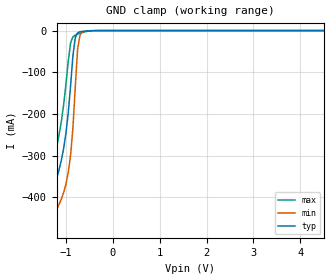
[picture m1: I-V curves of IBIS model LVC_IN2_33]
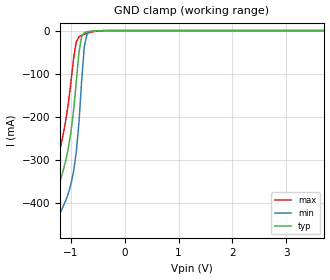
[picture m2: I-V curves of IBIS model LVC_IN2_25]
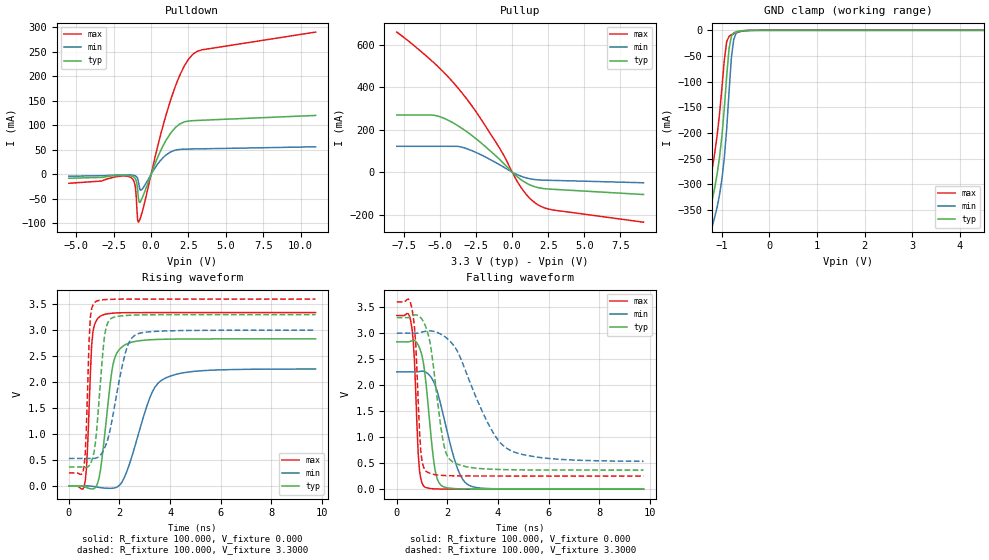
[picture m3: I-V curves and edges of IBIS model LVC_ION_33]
| NXP Semiconductors
| Logic Products Group
| IBIS model of 74LVC245A
|  OCTAL BUS TRANSCEIVER WITH DIRECTION PIN; 3-STATE; 5V TOLERANT
|[Packages]:
|[Package1]: SO 20-pin (D) Package ;
|[Package2]: SSOP 20-Pin Packages ;
|[Package3]: TSSOP 20-pin (PW) Package ;
|[Package4]: DHVQFN 20-pin (BQ) Package ;
[IBIS Ver]   3.2
[File Name]   lvc245a.ibs
[File Rev]   1.4
[Date]   06-Apr-2012
[Source]   File created from simulations by LPG
   NXP Semiconductors Nijmegen
[Notes]   V1.4   Ibis model.
| Remark:
| The Power Clamp curves have been omitted since there is no power clamp diode.
| Revision History
| Version Date   Author/ Description
|   Editor
| 1.0   1999   Initial Version
| 1.1   November 2001 RM   Revised for Ibis 3.2:
|   Added Model Spec and Model Selector
| 1.2   April   2002 RM   Corrected Model mapping in package models
| 1.3   November 2002 RM   Revised: Power Clamp curves omitted, constant
|   end points for Ground Clamp and V/t curves.
| 1.4   April   2012 RV   Updates pcakge models.
|   Added DHVQFN (BQ) package model
[Disclaimer]
   NXP Semiconductors warrants and represents that the IBIS model
   identified herein is owned by NXP Semiconductors (NXP). The
   model provided is not warranted as fully representing all of the
   operating characteristics and specifications of the semiconductor
   products to which the model relates.  Moreover, unless there is a
   signed, written agreement to the contrary, this IBIS model is
   furnished on an "as is" basis without support or warranty of any
   kind, either expressed or implied, regarding the use thereof, and
   NXP specifically disclaims all implied warranties of
   merchantability and fitness of the model for any purpose.
   NXP does not assume any liability arising out of the application
   or use of this IBIS model including infringement of patents and
   copyrights, nor does NXP convey any license under its patents and
   copyrights or the rights of others.
   NXP provides IBIS models as a service to our customers. You and
   your company shall not distribute, convey, sell, or give these models
   to anyone else without receiving prior written permission from
   NXP.
   NXP reserves the right to make changes without notice to these
   IBIS models to improve reliability, function, or design.
   Please be aware that your receipt and subsequent use of the IBIS
   information provided shall serve as acceptance of the terms and
   conditions of this agreement.  If you do not accept these terms,
   you should return or destroy the IBIS models and any other
   accompanying information immediately.
[Copyright]
   (C) Copyright 2012 NXP Semiconductors
   All rights reserved
|   Info for  SO 20-pin (D) Package
[Component]   74LVC245A_D
[Manufacturer]   NXP Semiconductors
[Package]
|   typ   min   max
R_pkg   1.303E-01   1.269E-01   1.360E-01
L_pkg   4.335E-09   3.559E-09   5.739E-09
C_pkg   8.078E-13   6.647E-13   1.016E-12
[Pin] signal_name   model_name   R_pin   L_pin   C_pin
   1   DIR   lvc_in2 1.359E-01   5.726E-09   1.016E-12
   2   A0   lvc_ion 1.318E-01   4.676E-09   8.893E-13
   3   A1   lvc_ion 1.290E-01   3.989E-09   7.599E-13
   4   A2   lvc_ion 1.277E-01   3.713E-09   7.096E-13
   5   A3   lvc_ion 1.269E-01   3.565E-09   6.651E-13
   6   A4   lvc_ion 1.269E-01   3.566E-09   6.652E-13
   7   A5   lvc_ion 1.278E-01   3.720E-09   7.096E-13
   8   A6   lvc_ion 1.291E-01   4.009E-09   7.592E-13
   9   A7   lvc_ion 1.319E-01   4.689E-09   8.893E-13
   10   GND   GND 1.359E-01   5.726E-09   1.016E-12
   11   B7   lvc_ion 1.360E-01   5.739E-09   1.015E-12
   12   B6   lvc_ion 1.319E-01   4.687E-09   8.894E-13
   13   B5   lvc_ion 1.289E-01   3.979E-09   7.598E-13
   14   B4   lvc_ion 1.277E-01   3.706E-09   7.097E-13
   15   B3   lvc_ion 1.269E-01   3.560E-09   6.648E-13
   16   B2   lvc_ion 1.269E-01   3.559E-09   6.647E-13
   17   B1   lvc_ion 1.277E-01   3.707E-09   7.096E-13
   18   B0   lvc_ion 1.290E-01   3.990E-09   7.589E-13
   19   OE#   lvc_in2 1.318E-01   4.674E-09   8.891E-13
   20   VCC   POWER 1.359E-01   5.719E-09   1.016E-12
|   Info for SSOP (DB) 20-Pin Packages
[Component]   74LVC245A_DB
[Manufacturer]   NXP Semiconductors
[Package]
|   typ   min   max
R_pkg   1.170E-01   9.466E-02   1.330E-01
L_pkg   2.881E-09   2.301E-09   3.694E-09
C_pkg   5.134E-13   4.076E-13   6.074E-13
[Pin] signal_name   model_name   R_pin   L_pin   C_pin
   1   DIR   lvc_in2 1.319E-01   3.694E-09   5.788E-13
   2   A0   lvc_ion 1.294E-01   3.215E-09   6.058E-13
   3   A1   lvc_ion 1.259E-01   2.779E-09   5.353E-13
   4   A2   lvc_ion 1.028E-01   2.436E-09   4.753E-13
   5   A3   lvc_ion 9.475E-02   2.308E-09   4.565E-13
   6   A4   lvc_ion 9.474E-02   2.307E-09   4.568E-13
   7   A5   lvc_ion 1.028E-01   2.433E-09   4.753E-13
   8   A6   lvc_ion 1.259E-01   2.774E-09   5.356E-13
   9   A7   lvc_ion 1.295E-01   3.206E-09   6.070E-13
   10   GND   GND 1.330E-01   3.679E-09   4.076E-13
   11   B7   lvc_ion 1.317E-01   3.678E-09   5.790E-13
   12   B6   lvc_ion 1.293E-01   3.209E-09   6.060E-13
   13   B5   lvc_ion 1.258E-01   2.758E-09   5.351E-13
   14   B4   lvc_ion 1.028E-01   2.427E-09   4.749E-13
   15   B3   lvc_ion 9.466E-02   2.301E-09   4.565E-13
   16   B2   lvc_ion 9.472E-02   2.307E-09   4.566E-13
   17   B1   lvc_ion 1.028E-01   2.434E-09   4.750E-13
   18   B0   lvc_ion 1.259E-01   2.769E-09   5.354E-13
   19   OE#   lvc_in2 1.296E-01   3.220E-09   6.074E-13
   20   VCC   POWER 1.329E-01   3.680E-09   4.076E-13
|   Info for  TSSOP 20-pin (PW) Package
[Component]   74LVC245A_PW
[Manufacturer]   NXP Semiconductors
[Package]
|   typ   min   max
R_pkg   8.765E-02   8.574E-02   9.134E-02
L_pkg   2.180E-09   1.913E-09   2.812E-09
C_pkg   3.300E-13   2.758E-13   4.019E-13
[Pin] signal_name   model_name   R_pin   L_pin   C_pin
   1   DIR   lvc_in2 9.132E-02   2.811E-09   4.003E-13
   2   A0   lvc_ion 8.924E-02   2.335E-09   3.938E-13
   3   A1   lvc_ion 8.600E-02   1.921E-09   2.996E-13
   4   A2   lvc_ion 8.597E-02   1.922E-09   2.800E-13
   5   A3   lvc_ion 8.576E-02   1.914E-09   2.764E-13
   6   A4   lvc_ion 8.574E-02   1.913E-09   2.767E-13
   7   A5   lvc_ion 8.595E-02   1.921E-09   2.803E-13
   8   A6   lvc_ion 8.594E-02   1.921E-09   2.995E-13
   9   A7   lvc_ion 8.925E-02   2.334E-09   3.943E-13
   10   GND   GND 9.130E-02   2.809E-09   4.019E-13
   11   B7   lvc_ion 9.134E-02   2.812E-09   4.002E-13
   12   B6   lvc_ion 8.925E-02   2.332E-09   3.937E-13
   13   B5   lvc_ion 8.600E-02   1.920E-09   2.993E-13
   14   B4   lvc_ion 8.597E-02   1.921E-09   2.794E-13
   15   B3   lvc_ion 8.576E-02   1.914E-09   2.758E-13
   16   B2   lvc_ion 8.574E-02   1.913E-09   2.762E-13
   17   B1   lvc_ion 8.596E-02   1.921E-09   2.798E-13
   18   B0   lvc_ion 8.595E-02   1.921E-09   2.993E-13
   19   OE#   lvc_in2 8.925E-02   2.331E-09   3.936E-13
   20   VCC   POWER 9.134E-02   2.812E-09   4.003E-13
|   Info for  DHVQFN 20-pin (BQ) Package
[Component]   74LVC245A_BQ
[Manufacturer]   NXP Semiconductors
[Package]
|   typ   min   max
R_pkg   9.848E-02   7.975E-02   1.188E-01
L_pkg   1.518E-09   1.230E-09   1.831E-09
C_pkg   2.028E-13   1.724E-13   2.307E-13
[Pin] signal_name   model_name   R_pin   L_pin   C_pin
   1   DIR   lvc_in2 1.187E-01   1.831E-09   2.169E-13
   2   A0   lvc_ion 1.188E-01   1.831E-09   2.166E-13
   3   A1   lvc_ion 9.536E-02   1.470E-09   2.030E-13
   4   A2   lvc_ion 7.977E-02   1.230E-09   1.851E-13
   5   A3   lvc_ion 7.977E-02   1.230E-09   1.851E-13
   6   A4   lvc_ion 7.977E-02   1.230E-09   1.849E-13
   7   A5   lvc_ion 7.977E-02   1.230E-09   1.851E-13
   8   A6   lvc_ion 9.536E-02   1.470E-09   2.028E-13
   9   A7   lvc_ion 1.188E-01   1.830E-09   2.300E-13
   10   GND   GND 1.188E-01   1.830E-09   2.307E-13
   11   B7   lvc_ion 1.188E-01   1.831E-09   2.173E-13
   12   B6   lvc_ion 1.187E-01   1.831E-09   2.168E-13
   13   B5   lvc_ion 9.534E-02   1.471E-09   1.902E-13
   14   B4   lvc_ion 7.975E-02   1.231E-09   1.724E-13
   15   B3   lvc_ion 7.977E-02   1.230E-09   1.857E-13
   16   B2   lvc_ion 7.977E-02   1.230E-09   1.850E-13
   17   B1   lvc_ion 7.975E-02   1.230E-09   1.849E-13
   18   B0   lvc_ion 9.535E-02   1.470E-09   2.029E-13
   19   OE#   lvc_in2 1.188E-01   1.830E-09   2.301E-13
   20   VCC   POWER 1.188E-01   1.830E-09   2.299E-13
[Model Selector]   lvc_in2
LVC_IN2_33   3.3V-Vcc input model
LVC_IN2_25   2.5V-Vcc input model
[Model Selector]   lvc_ion
LVC_ION_33   3.3V-Vcc I/O model, non-inverting
LVC_ION_25   2.5V-Vcc I/O model, non-inverting
| Models and submodels in the file (4): LVC_IN2_33 (Input), LVC_IN2_25 (Input), LVC_ION_33 (I/O), LVC_ION_25 (I/O)
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| Remark: If your software does not support the Model Selector
|   Please comment out the lines of the Model Selector, which
|   contain the name of the Model, except the one you want to use.
|   Model LVC_IN2_33
[Model]   LVC_IN2_33
Model_type   Input
Vinl =   0.8000V
Vinh =   2.0000V
C_comp   2.78pF   1.99pF   3.72pF
[Model Spec]
| Note: The input and output voltage ratings may be exceeded if the input and
|   output current ratings are observed (please refer to the data sheet)
|   Subparameter   typ   min   max
| Thresholds
Vinh   2.0   NA   NA
Vinl   0.8   NA   NA
| Overshoot
S_overshoot_high   6.5   6.5   6.5   | Static overshoot
S_overshoot_low   -0.5   -0.5   -0.5
D_overshoot_high   7.2   7.2   7.2   | Dynamic overshoot
D_overshoot_low   -0.95   -0.9   -1.0
D_overshoot_time   3n   3n   3n
|Ambient temperature:   25.0000   85.0000   -40.0000
[Temperature Range]   40.0000   100.0000   -25.0000
[Voltage Range]   3.3000V   3.0000V   3.6000V
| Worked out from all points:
|   GND clamp passes 1 mA (typ) near -0.57 V on its own axis
|Process Range   nominal   slow   fast
[GND_clamp]
| voltage   I(typ)   I(min)   I(max)
-5.5V     -4.567A    -4.624A    -4.51A
-1.45V    -555.2mA   -621.5mA   -488.4mA
-1.35V    -461.8mA   -528.7mA   -394.3mA
-1.3V     -417.5mA   -485mA     -349.4mA
-1.1V     -312.4mA   -404.8mA   -219.8mA
-950mV    -197.3mA   -340.4mA   -73.13mA
-900mV    -132mA     -298.5mA   -29.44mA
-850mV    -59.79mA   -233mA     -14.94mA
-800mV    -16.87mA   -135mA     -10.93mA
-750mV    -5.479mA   -44.49mA   -8.487mA
-700mV    -2.88mA    -11.01mA   -6.407mA
5.5V      1.567nA    9.324nA    202.5pA
|   Model LVC_IN2_25
[Model]   LVC_IN2_25
Model_type   Input
Vinl =   0.7000V
Vinh =   1.7000V
C_comp   2.84pF   2.10pF   3.71pF
[Model Spec]
| Note: The input and output voltage ratings may be exceeded if the input and
|   output current ratings are observed (please refer to the data sheet)
|   Subparameter   typ   min   max
| Thresholds
Vinh   1.7   NA   NA
Vinl   0.7   NA   NA
| Overshoot
S_overshoot_high   6.5   6.5   6.5   | Static overshoot
S_overshoot_low   -0.5   -0.5   -0.5
D_overshoot_high   7.2   7.2   7.2   | Dynamic overshoot
D_overshoot_low   -0.95   -0.9   -1.0
D_overshoot_time   3n   3n   3n
|Ambient temperature:   25.0000   85.0000   -40.0000
[Temperature Range]   35.0000   95.0000   -30.0000
[Voltage Range]   2.5000V   2.3000V   2.7000V
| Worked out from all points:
|   GND clamp passes 1 mA (typ) near -0.57 V on its own axis
|Process Range   nominal   slow   fast
[GND_clamp]
| voltage   I(typ)   I(min)   I(max)
-5.5V     -4.558A    -4.615A    -4.502A
-1.45V    -549mA     -615mA     -482.5mA
-1.35V    -455.6mA   -522.2mA   -388.4mA
-1.3V     -411.3mA   -478.6mA   -343.5mA
-1.1V     -304mA     -396mA     -212mA
-950mV    -185.1mA   -326.6mA   -65.02mA
-900mV    -119.1mA   -281.8mA   -26.08mA
-850mV    -50.24mA   -213.2mA   -14.46mA
-800mV    -13.81mA   -116mA     -10.88mA
-750mV    -4.865mA   -35.92mA   -8.446mA
-700mV    -2.732mA   -8.828mA   -6.333mA
5.5V      922.9pA    6.4nA      86.94pA
|   Model LVC_ION_33
[Model]   LVC_ION_33
Model_type   I/O
Polarity   Non-Inverting
Enable   Active-Low
Vinl  =  0.8000V
Vinh  =  2.0000V
Vmeas =  1.5000V
Cref  = 50.0000pF
Rref  =  0.5000k
Vref  =  0.000V
C_comp   3.67pF   3.24pF   4.23pF
[Model Spec]
| Note: The input and output voltage ratings may be exceeded if the input and
|   output current ratings are observed (please refer to the data sheet)
|   Subparameter   typ   min   max
| Overshoot
S_overshoot_high   6.5   6.5   6.5   | Static overshoot
S_overshoot_low   -0.5   -0.5   -0.5
D_overshoot_high   7.2   7.2   7.2   | Dynamic overshoot
D_overshoot_low   -0.95   -0.9   -1.0
D_overshoot_time   3n   3n   3n
| Timing Thresholds
Vmeas   1.5   1.5   1.5
|Ambient temperature:   25.0000   85.0000   -40.0000
[Temperature Range]   40.0000   100.0000   -25.0000
[Voltage Range]   3.3000V   3.0000V   3.6000V
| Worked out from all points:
|   slope of the pulldown table from 0 to 0.495 V, typ, clamps not added: 12.8 ohm
|   slope of the pullup table from 0 to 0.495 V, typ, clamps not added: 16.7 ohm
|   GND clamp passes 1 mA (typ) near -0.57 V on its own axis
|   rising waveform, R_fixture 100.000, V_fixture 0.000: 20-80 % time 400ps typ, 877ps min, 167ps max; typ from 0 V to 2.83 V
|   rising waveform, R_fixture 100.000, V_fixture 3.3000: 20-80 % time 297ps typ, 599ps min, 140ps max; typ from 0.367 V to 3.3 V
|   falling waveform, R_fixture 100.000, V_fixture 0.000: 20-80 % time 354ps typ, 719ps min, 176ps max; typ from 2.83 V to 0 V
|   falling waveform, R_fixture 100.000, V_fixture 3.3000: 20-80 % time 471ps typ, 1.35ns min, 197ps max; typ from 3.3 V to 0.367 V
|Process Range   nominal   slow   fast
[Pulldown]
| voltage   I(typ)   I(min)   I(max)
-5.5V     -7.981mA   -3.814mA   -18.26mA
-1.35V    -3.285mA   -1.337mA   -6.644mA
-1.05V    -9.131mA   -3.158mA   -26.89mA
-900mV    -31.33mA   -8.405mA   -93.71mA
-850mV    -48.34mA   -14.32mA   -97.69mA
-800mV    -56.89mA   -23.68mA   -95.44mA
-650mV    -51.7mA    -31.9mA    -82.65mA
500mV     38.92mA    23.46mA    64.5mA
1.3V      83.8mA     45.64mA    151.3mA
2.2V      106.9mA    51.35mA    220.1mA
2.8V      109.6mA    51.79mA    245.4mA
11V       120.3mA    56.22mA    290.4mA
[Pullup]
| voltage   I(typ)   I(min)   I(max)
-8V       269.1mA    121.8mA    660.4mA
-5.4V     268mA      121.8mA    514mA
-4.4V     243.3mA    121.8mA    446.3mA
-3.6V     211.5mA    119.5mA    383.9mA
-2.4V     151.5mA    89.4mA     274mA
-800mV    55.11mA    31.81mA    104.4mA
600mV     -35.22mA   -19.02mA   -71.23mA
1V        -52.59mA   -27.82mA   -107.4mA
1.6V      -69.81mA   -35.37mA   -146mA
2.2V      -77.8mA    -37.89mA   -167.8mA
2.8V      -81.05mA   -39.02mA   -178.1mA
9.1V      -105.6mA   -50.26mA   -236.2mA
[GND_clamp]
| voltage   I(typ)   I(min)   I(max)
-5.5V     -4.552A    -4.581A    -4.529A
-1.35V    -436.9mA   -483.2mA   -382.8mA
-1.3V     -392.7mA   -439.6mA   -337.9mA
-1.2V     -328.9mA   -381mA     -268.2mA
-1.05V    -247.4mA   -320.5mA   -163.3mA
-950mV    -153.3mA   -249mA     -58.72mA
-900mV    -90.37mA   -192.9mA   -22.55mA
-850mV    -36.04mA   -120.8mA   -11.79mA
-800mV    -11.48mA   -52.5mA    -8.579mA
-750mV    -4.615mA   -17.21mA   -6.53mA
-700mV    -2.665mA   -5.464mA   -4.804mA
5.5V      991.5pA    8.054nA    37.33pA
[Ramp]
| variable   typ   min   max
dV/dt_r   1.700V/400.499ps   1.352V/877.029ps   2.004V/166.817ps
dV/dt_f   1.760V/471.272ps   1.479V/1.352ns   2.008V/196.882ps
R_load = 100.000
[Rising Waveform]
R_fixture   = 100.000
V_fixture   = 0.000
V_fixture_min = 0.000
V_fixture_max = 0.000
| time   V(typ)   V(min)   V(max)
0s        66.72pV    2.831nV    5.104pV
650ps     -20.04mV   787uV      106.7mV
750ps     -38.64mV   1.118mV    865.9mV
900ps     -55.77mV   -3.748mV   2.705V
1.25ns    312.5mV    -31.4mV    3.272V
1.75ns    2.35V      -42.26mV   3.329V
2.2ns     2.713V     172.1mV    3.337V
3.2ns     2.816V     1.7V       3.34V
3.7ns     2.825V     2.047V     3.34V
9.75ns    2.833V     2.253V     3.34V
[Rising Waveform]
R_fixture   = 100.000
V_fixture   = 3.3000
V_fixture_min = 3.0000
V_fixture_max = 3.6000
| time   V(typ)   V(min)   V(max)
0s        366.8mV    531.4mV    252.7mV
600ps     358.5mV    532mV      365.8mV
650ps     356.5mV    532.2mV    639.8mV
850ps     427.8mV    529.9mV    3.253V
1.05ns    835.2mV    534.7mV    3.548V
1.4ns     2.845V     722.3mV    3.588V
1.7ns     3.235V     1.252V     3.596V
2.25ns    3.284V     2.593V     3.599V
2.7ns     3.293V     2.925V     3.6V
9.75ns    3.3V       3V         3.6V
[Falling Waveform]
R_fixture   = 100.000
V_fixture   = 0.000
V_fixture_min = 0.000
V_fixture_max = 0.000
| time   V(typ)   V(min)   V(max)
0s        2.833V     2.255V     3.34V
550ps     2.845V     2.255V     3.241V
700ps     2.855V     2.254V     2.457V
900ps     2.715V     2.264V     349.4mV
1.1ns     2.269V     2.259V     43.59mV
1.5ns     408.7mV    2.02V      5.848mV
1.8ns     57.88mV    1.501V     2.421mV
2.4ns     8.231mV    399.2mV    587.4uV
2.95ns    3.443mV    54.81mV    163.2uV
9.75ns    -682.6nV   100.1uV    3.08pV
[Falling Waveform]
R_fixture   = 100.000
V_fixture   = 3.3000
V_fixture_min = 3.0000
V_fixture_max = 3.6000
| time   V(typ)   V(min)   V(max)
0s        3.3V       3V         3.6V
600ps     3.326V     2.999V     3.473V
750ps     3.353V     2.998V     2.782V
950ps     3.295V     3.014V     728.3mV
1.15ns    3.116V     3.038V     345.8mV
1.35ns    2.716V     3.043V     298.4mV
1.85ns    878.2mV    2.95V      263.4mV
2.2ns     528.7mV    2.793V     257.4mV
4.4ns     374.3mV    769.3mV    252.8mV
9.75ns    366.9mV    536.4mV    252.7mV
